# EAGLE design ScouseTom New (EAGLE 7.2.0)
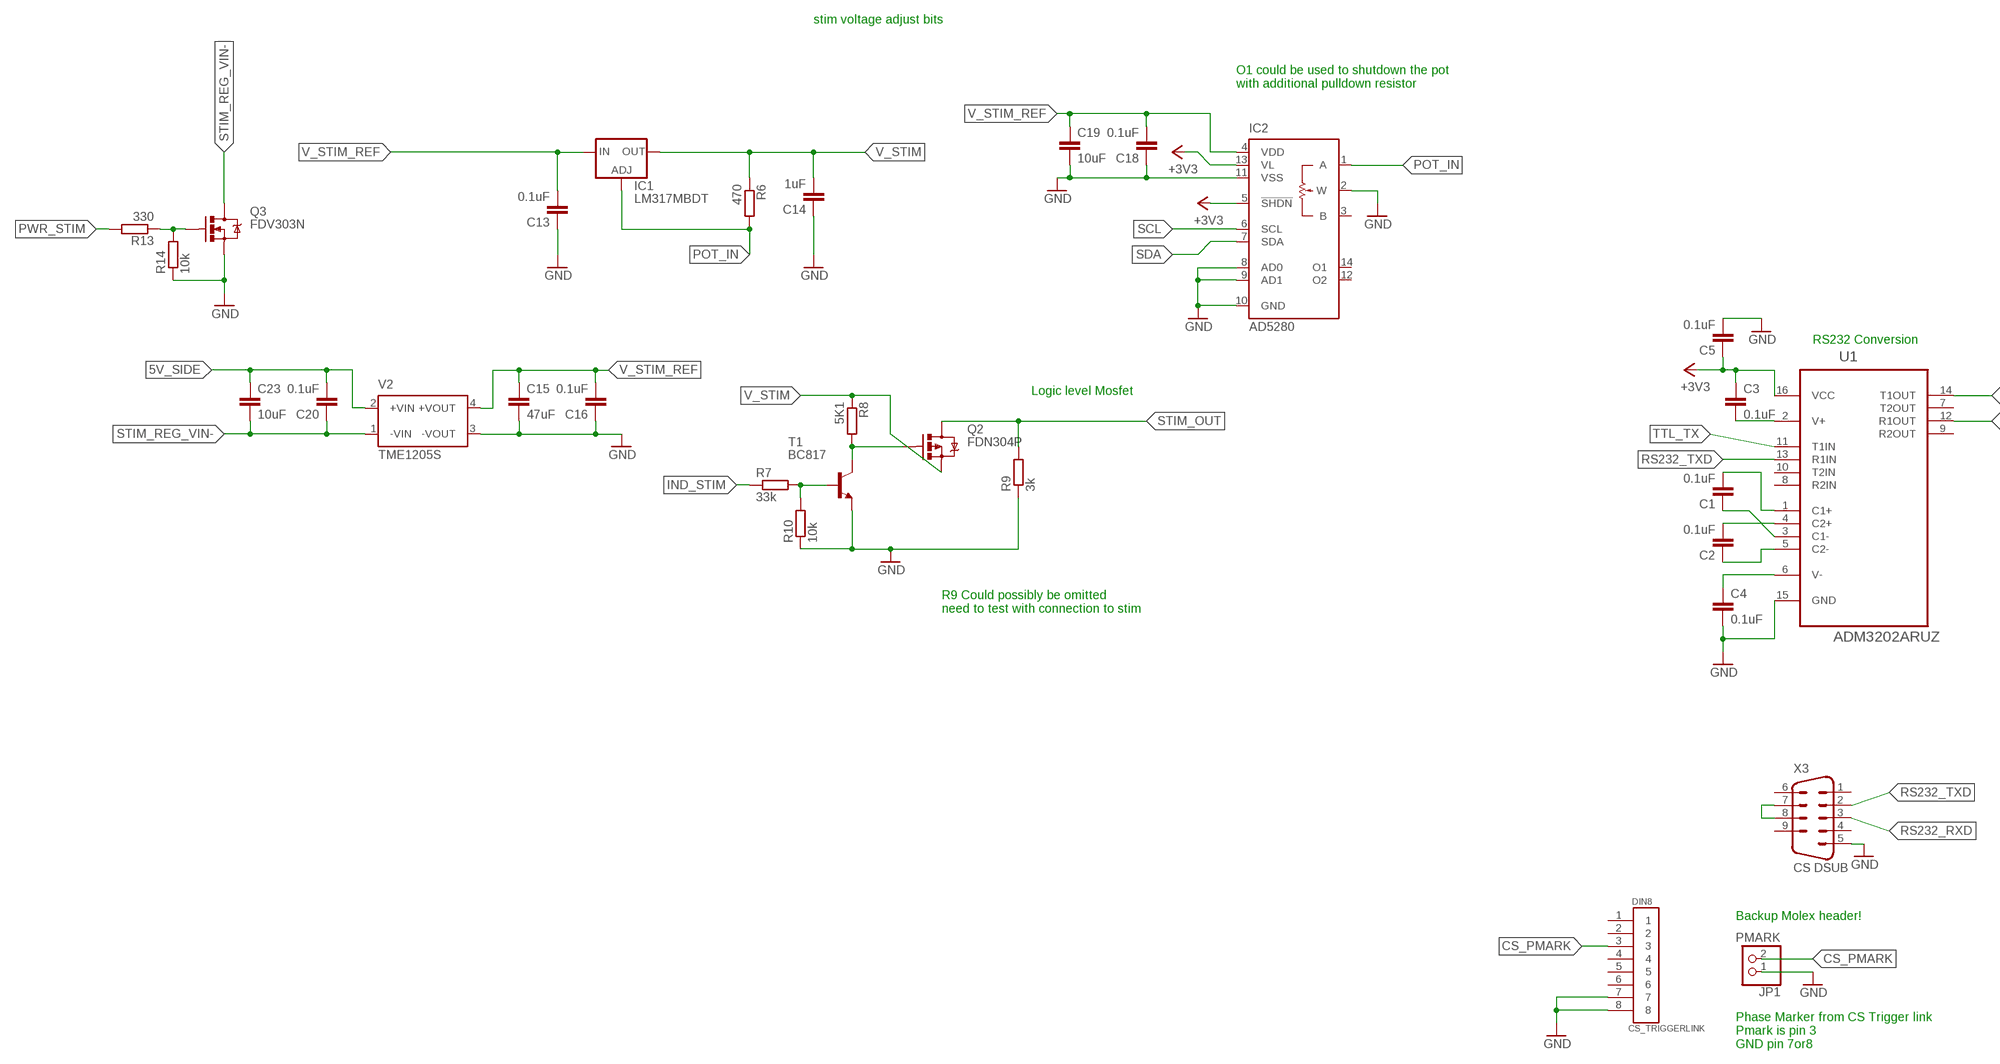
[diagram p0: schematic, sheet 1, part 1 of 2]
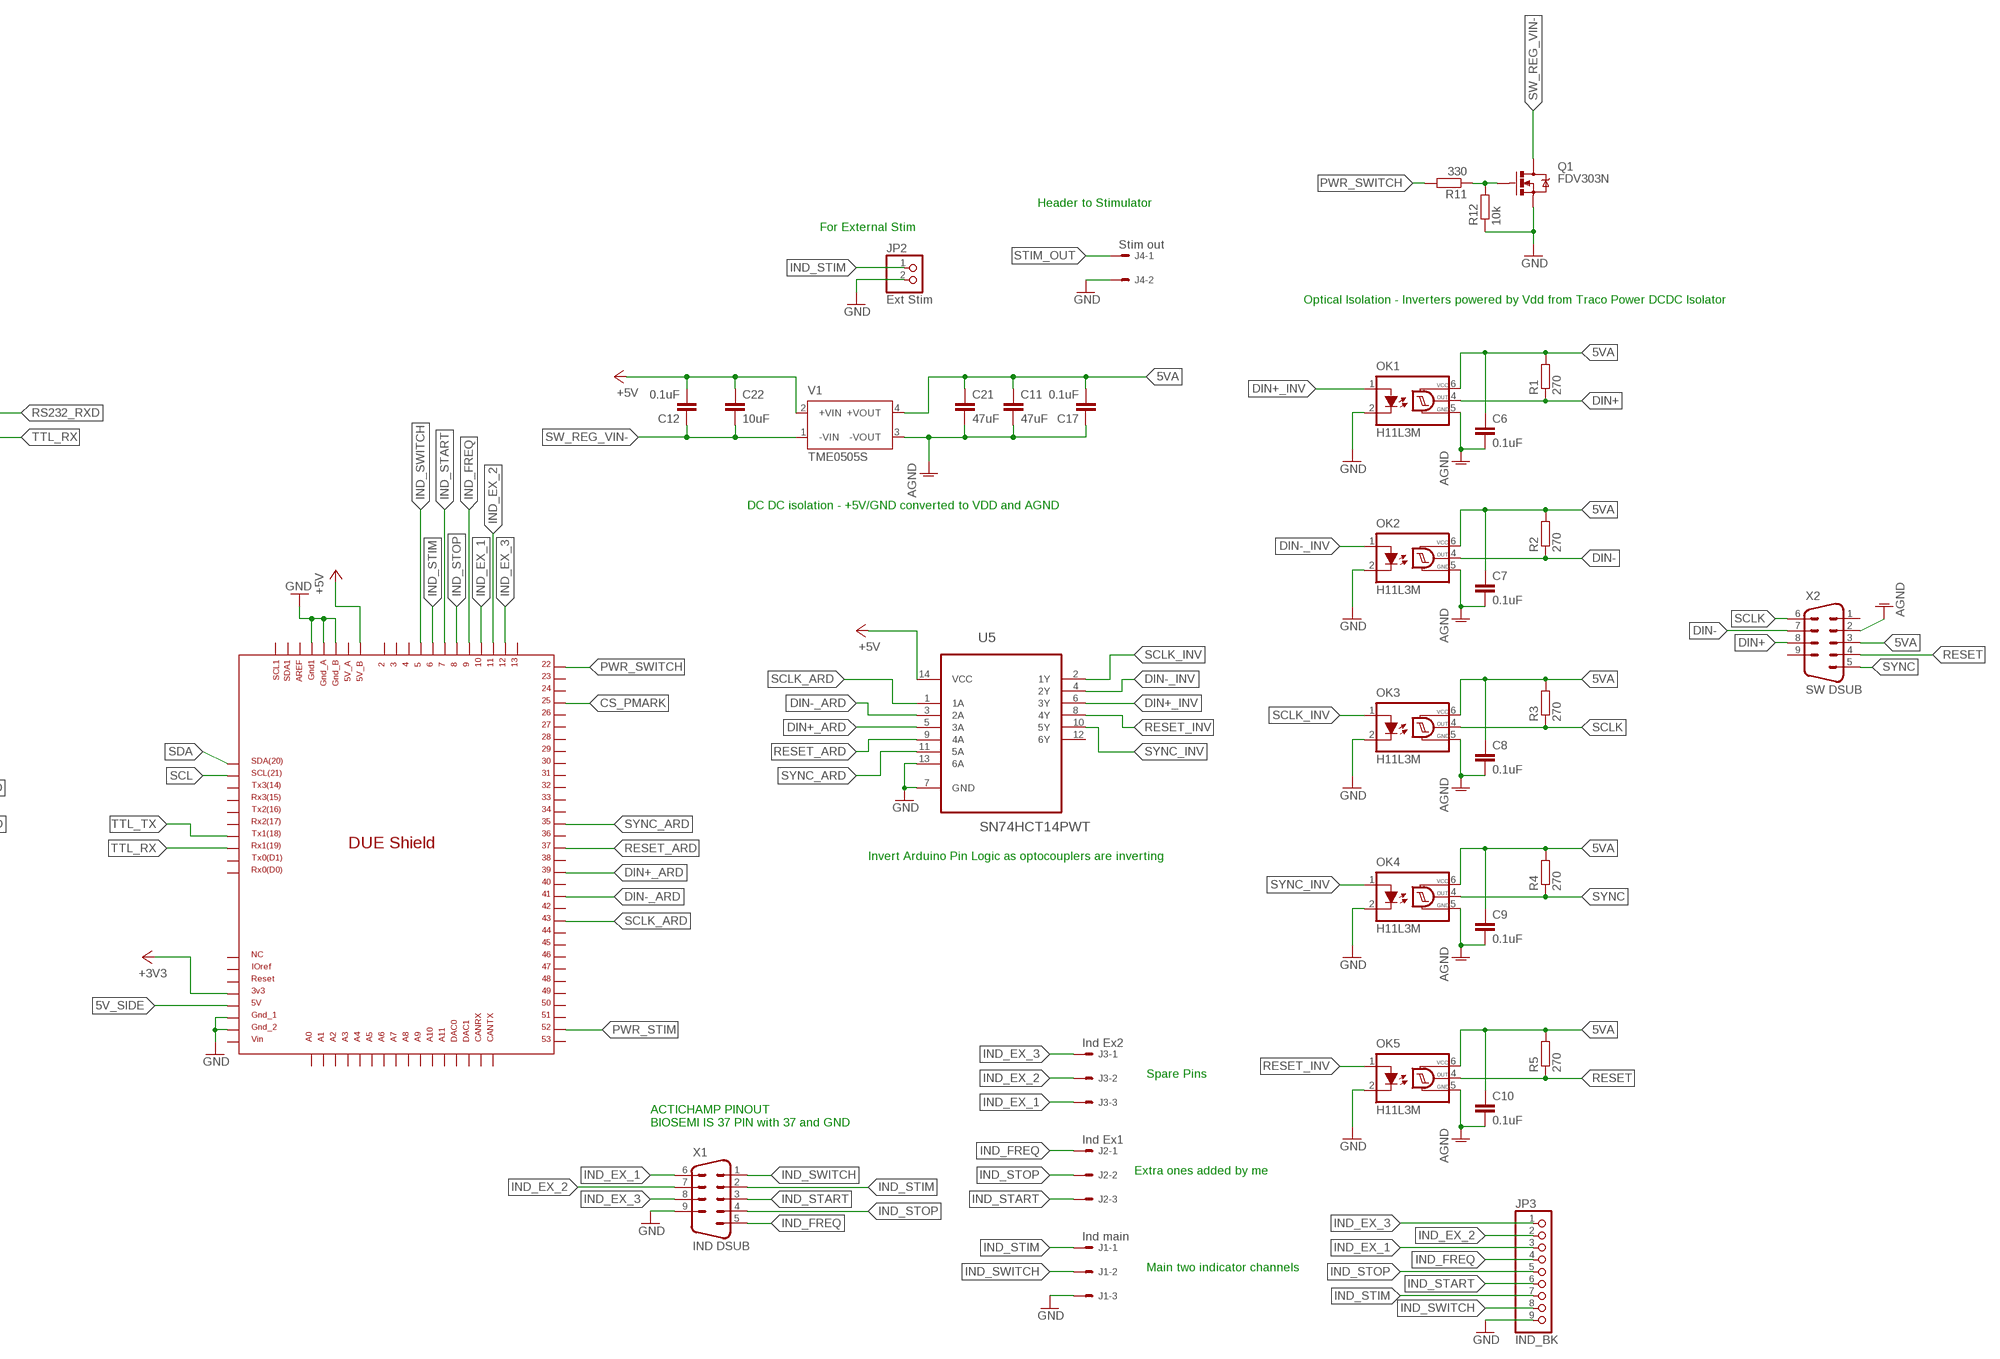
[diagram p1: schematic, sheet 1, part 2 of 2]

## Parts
C1  0.1uF  C-EUC0805  [C0805]
C2  0.1uF  C-EUC0805  [C0805]
C3  0.1uF  C-EUC0805  [C0805]
C4  0.1uF  C-EUC0805  [C0805]
C5  0.1uF  C-EUC0805  [C0805]
C6  0.1uF  C-EUC0805  [C0805]
C7  0.1uF  C-EUC0805  [C0805]
C8  0.1uF  C-EUC0805  [C0805]
C9  0.1uF  C-EUC0805  [C0805]
C10  0.1uF  C-EUC0805  [C0805]
C11  47uF  C-EUC0805  [C0805]
C12  0.1uF  C-EUC0805  [C0805]
C13  0.1uF  C-EUC0805  [C0805]
C14  1uF  C-EUC0805  [C0805]
C15  47uF  C-EUC0805  [C0805]
C16  0.1uF  C-EUC0805  [C0805]
C17  0.1uF  C-EUC0805  [C0805]
C18  0.1uF  C-EUC0805  [C0805]
C19  10uF  C-EUC0805  [C0805]
C20  0.1uF  C-EUC0805  [C0805]
C21  47uF  C-EUC0805  [C0805]
C22  10uF  C-EUC0805  [C0805]
C23  10uF  C-EUC0805  [C0805]
DIN8  CS_TRIGGERLINK  DIN8  [DIN8]
DUE  DUE(NOMID)  [DUE(NOMID)]
IC1  LM317MBDT  [DPACK]
IC2  AD5280  [TSSOP14]
J1  Ind main  22-27-2031-03  [6410-03]
J2  Ind Ex1  22-27-2031-03  [6410-03]
J3  Ind Ex2  22-27-2031-03  [6410-03]
J4  Stim out  22-27-2021-02  [6410-02]
JP1  PMARK  PINHD-1X2  [1X02]
JP2  Ext Stim  PINHD-1X2  [1X02]
JP3  IND_BK  PINHD-1X9  [1X09]
OK1  H11L3M  [DIL06]
OK2  H11L3M  [DIL06]
OK3  H11L3M  [DIL06]
OK4  H11L3M  [DIL06]
OK5  H11L3M  [DIL06]
Q1  FDV303N  MOSFET-NCHANNEL2N7002PW  [SOT323]
Q2  FDN304P  MOSFET-PCHANNEL  [SOT23-3]
Q3  FDV303N  MOSFET-NCHANNEL2N7002PW  [SOT323]
R1  270  R-EU_R0805  [R0805]
R2  270  R-EU_R0805  [R0805]
R3  270  R-EU_R0805  [R0805]
R4  270  R-EU_M0805  [M0805]
R5  270  R-EU_M0805  [M0805]
R6  470  R-EU_R0805  [R0805]
R7  33k  R-EU_R0805  [R0805]
R8  5K1  R-EU_R0805  [R0805]
R9  3k  R-EU_R0805  [R0805]
R10  10k  R-EU_R0805  [R0805]
R11  330  R-EU_R0805  [R0805]
R12  10k  R-EU_R0805  [R0805]
R13  330  R-EU_R0805  [R0805]
R14  10k  R-EU_R0805  [R0805]
T1  BC817  BC817-40SMD  [SOT23-BEC]
U1  ADM3202ARUZ  [SOP65P640X120-16N]
U5  SN74HCT14PWT  [SOP65P640X120-14N]
V1  TME0505S  [TME]
V2  TME1205S  [TME]
X1  IND DSUB  DSUB9RA  [DSUB9]
X2  SW DSUB  DSUB9RA  [DSUB9]
X3  CS DSUB  DSUB9RA  [DSUB9]

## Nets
5V_SIDE: C20.2 C23.1 DUE.5V V2.2(+VIN)
5VA: C6.1 C7.1 C8.1 C9.1 C10.1 C11.1 C17.2 C21.1 OK1.6(VCC) OK2.6(VCC) OK3.6(VCC) OK4.6(VCC) OK5.6(VCC) R1.2 R2.2 R3.2 R4.2 R5.2 V1.4(+VOUT) X2.3
+3V3: C3.1 C5.1 DUE.3V3 IC2.5(!SHDN) IC2.13(VL) U1.16(VCC)
+5V: C12.2 C22.1 DUE.5V_B U5.14(VCC) V1.2(+VIN)
AGND: C6.2 C7.2 C8.2 C9.2 C10.2 C11.2 C17.1 C21.2 OK1.5(GND) OK2.5(GND) OK3.5(GND) OK4.5(GND) OK5.5(GND) V1.3(-VOUT) X2.2
CS_PMARK: DIN8.3 DUE.25 JP1.2
DIN+: OK1.4(OUT) R1.1 X2.8
DIN+_ARD: DUE.39 U5.5(3A)
DIN+_INV: OK1.1(A) U5.6(3Y)
DIN-: OK2.4(OUT) R2.1 X2.7
DIN-_ARD: DUE.41 U5.3(2A)
DIN-_INV: OK2.1(A) U5.4(2Y)
GND: C4.2 C5.2 C13.1 C14.1 C15.2 C16.1 C18.1 C19.2 DIN8.7 DIN8.8 DUE.GND1 DUE.GND_1 DUE.GND_2 DUE.GND_A DUE.GND_B IC2.2(W) IC2.8(AD0) IC2.9(AD1) IC2.10(GND) IC2.11(VSS) J1.3 J4.2 JP1.1 JP2.2 JP3.9 OK1.2(C) OK2.2(C) OK3.2(C) OK4.2(C) OK5.2(C) Q1.2(S) Q3.2(S) R9.1 R10.1 R12.1 R14.1 T1.E U1.15(GND) U5.7(GND) U5.13(6A) V2.3(-VOUT) X1.9 X3.5
IND_EX_1: DUE.10 J3.3 JP3.3 X1.6
IND_EX_2: DUE.11 J3.2 JP3.2 X1.7
IND_EX_3: DUE.12 J3.1 JP3.1 X1.8
IND_FREQ: DUE.9 J2.1 JP3.4 X1.5
IND_START: DUE.7 J2.3 JP3.6 X1.3
IND_STIM: DUE.6 J1.1 JP2.1 JP3.7 R7.1 X1.2
IND_STOP: DUE.8 J2.2 JP3.5 X1.4
IND_SWITCH: DUE.5 J1.2 JP3.8 X1.1
N$1: R7.2 R10.2 T1.B
N$2: Q1.1(G) R11.1 R12.2
N$3: Q2.1(G) R8.2 T1.C
N$4: X3.7 X3.8
N$5: Q3.1(G) R13.1 R14.2
N$22: C1.2 U1.1(C1+)
N$23: C1.1 U1.3(C1-)
N$24: C2.2 U1.4(C2+)
N$25: C2.1 U1.5(C2-)
N$26: C3.2 U1.2(V+)
N$27: C4.1 U1.6(V-)
POT_IN: IC1.1(ADJ) IC2.1(A) R6.2
PWR_STIM: DUE.52 R13.2
PWR_SWITCH: DUE.22 R11.2
RESET: OK5.4(OUT) R5.1 X2.4
RESET_ARD: DUE.37 U5.9(4A)
RESET_INV: OK5.1(A) U5.8(4Y)
RS232_RXD: U1.14(T1OUT) X3.3
RS232_TXD: U1.13(R1IN) X3.2
SCL: DUE.SCL IC2.6(SCL)
SCLK: OK3.4(OUT) R3.1 X2.6
SCLK_ARD: DUE.43 U5.1(1A)
SCLK_INV: OK3.1(A) U5.2(1Y)
SDA: DUE.SDA IC2.7(SDA)
STIM_OUT: J4.1 Q2.3(D) R9.2
STIM_REG_VIN-: C20.1 C23.2 Q3.3(D) V2.1(-VIN)
SW_REG_VIN-: C12.1 C22.2 Q1.3(D) V1.1(-VIN)
SYNC: OK4.4(OUT) R4.1 X2.5
SYNC_ARD: DUE.35 U5.11(5A)
SYNC_INV: OK4.1(A) U5.10(5Y)
TTL_RX: DUE.RX1 U1.12(R1OUT)
TTL_TX: DUE.TX1 U1.11(T1IN)
V_STIM: C14.2 IC1.4(OUT) Q2.2(S) R6.1 R8.1
V_STIM_REF: C13.2 C15.1 C16.2 C18.2 C19.1 IC1.3(IN) IC2.4(VDD) V2.4(+VOUT)
Unconnected: DIN8.1 DIN8.2 DIN8.4 DIN8.5 DIN8.6 DUE.2 DUE.3 DUE.4 DUE.5V_A DUE.13 DUE.23 DUE.24 DUE.26 DUE.27 DUE.28 DUE.29 DUE.30 DUE.31 DUE.32 DUE.33 DUE.34 DUE.36 DUE.38 DUE.40 DUE.42 DUE.44 DUE.45 DUE.46 DUE.47 DUE.48 DUE.49 DUE.50 DUE.51 DUE.53 DUE.A0 DUE.A1 DUE.A2 DUE.A3 DUE.A4 DUE.A5 DUE.A6 DUE.A7 DUE.A8 DUE.A9 DUE.A10 DUE.A11 DUE.AREF DUE.CANRX DUE.CANTX DUE.DAC0 DUE.DAC1 DUE.IOREF DUE.NC DUE.RESET DUE.RX0 DUE.RX2 DUE.RX3 DUE.SCL1 DUE.SDA1 DUE.TX0 DUE.TX2 DUE.TX3 DUE.VIN IC2.3(B) IC2.12(O2) IC2.14(O1) U1.7(T2OUT) U1.8(R2IN) U1.9(R2OUT) U1.10(T2IN) U5.12(6Y) X2.1 X2.9 X3.1 X3.4 X3.6 X3.9

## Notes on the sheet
- stim voltage adjust bits
- O1 could be used to shutdown the pot
  with additional pulldown resistor
- Header to Stimulator
- For External Stim
- Optical Isolation - Inverters powered by Vdd from Traco Power DCDC Isolator
- RS232 Conversion
- Logic level Mosfet
- DC DC isolation - +5V/GND converted to VDD and AGND
- R9 Could possibly be omitted
  need to test with connection to stim
- Invert Arduino Pin Logic as optocouplers are inverting
- Backup Molex header!
- Phase Marker from CS Trigger link
  Pmark is pin 3
  GND pin 7or8
- Spare Pins
- ACTICHAMP PINOUT
  BIOSEMI IS 37 PIN with 37 and GND
- Extra ones added by me
- Main two indicator channels

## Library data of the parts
C1-C23 = resistor:C-EU: CAPACITOR, European symbol
DIN8 = mini din 8 james:DIN8
DUE = DUElib130425_JAMES:DUE(NOMID)
IC1 = v-reg:LM317?*: 500 mA Adjustable Output Positive Voltage Regulator Source: http://www.onsemi.co.jp .. LM317M-D.PDF
IC2 = analog-devices:AD5280: Single +15 V/±5 V, 256-Position, I2C-Compatible Digital Potentiometer Source: http://www.analog.com/static/imported-files/data_sheets/AD5280_5282.pdf; MF: ALTERA CORPORATION; MPN: AD5280BRUZ20; OC_FARNELL: 1464325; OC_NEWARK: 59K3840
J1-J3 = con-molex:22-?-03: CONNECTOR wire to board 2.54 mm (.1 inch) pitch header; OC_FARNELL: unknown; OC_NEWARK: unknown
J4 = con-molex:22-?-02: CONNECTOR; OC_FARNELL: unknown; OC_NEWARK: unknown
JP1 JP2 = pinhead:PINHD-1X2: PIN HEADER
JP3 = pinhead:PINHD-1X9: PIN HEADER
OK1-OK5 = optocoupler:H11L*M: 6-Pin DIP Optocoupler Source: http://www.fairchildsemi.com/ds/H1/H11L2-M.pdf; MF: FAIRCHILD SEMICONDUCTOR; MPN: H11L3-M; OC_FARNELL: 1021233; OC_NEWARK: 72K8646
Q1 Q3 = SparkFun-DiscreteSemi:MOSFET-NCHANNEL: Common NMOSFET Parts MFG P/NStore IDProd ID FDD8780TRANS-09984 SI7820DNTRANS-11055 FDS6630AIC-08089 2N7002PWTRANS-11151 FQP30N06L COM-10213TRANS-10060 BSS123LT1GTRANS-08345 BSS138TRANS-00830 BS170 2N7000; PROD_ID: TRANS-11151
Q2 = SparkFun-DiscreteSemi:MOSFET-PCHANNEL: Generic PMOSFET IRLML2244 - TRANS-11153 (SOT-23 -20V -4.3A) (1.Gate 2.Source 3.Drain) FQP27P06 - COM-10349 (TO-220 -60V -27A) (1.Gate 2.Source 3.Drain); PROD_ID: TRANS-08285
R1-R14 = resistor:R-EU_: RESISTOR, European symbol
T1 = transistor-npn:BC817*: NPN Transistor
U1 = Analog Devices_By_element14_Batch_1:ADM3202ARUZ: Low Power, 3.3 V, RS-232 Line Drivers/Receivers; MPN: ADM3202ARUZ; OC_FARNELL: 9425586; OC_NEWARK: 59K2064; PACKAGE: TSSOP-16; SUPPLIER: Analog Devices
U5 = untitled:SN74HCT14PWT: QUADRUPLE FET BUS SWITCH 2.5-V/3.3-V LOW-VOLTAGE BUS SWITCH WITH 5-V-TOLERANT LEVEL SHIFTER; MPN: SN74HCT14PWT; OC_FARNELL: 1236233; OC_NEWARK: 13M5201; PACKAGE: TSSOP-14; SUPPLIER: Texas Instruments
V1 = traco-electronic:TME?*: DC/DC Converter TME Series 1 Watt Source: www.tracopower.com .. tme.pdf; MPN: TME 0505S; OC_FARNELL: 1007538; OC_NEWARK: 51R5321
V2 = traco-electronic:TME?*: DC/DC Converter TME Series 1 Watt Source: www.tracopower.com .. tme.pdf; MPN: TME 1205S; OC_FARNELL: 1007542; OC_NEWARK: 51R5325
X1-X3 = DSUBJAMES:DSUB9RA

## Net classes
1 power: width 0.61 mm, drill 0.61 mm, clearance 0.254 mm
2 gnd: width 0.305 mm, drill 0.559 mm, clearance 0.254 mm
3 usbvcc: width 0.508 mm, drill 0.61 mm, clearance 0.254 mm
4 aref: width 0.406 mm, drill 0.61 mm, clearance 0.254 mm

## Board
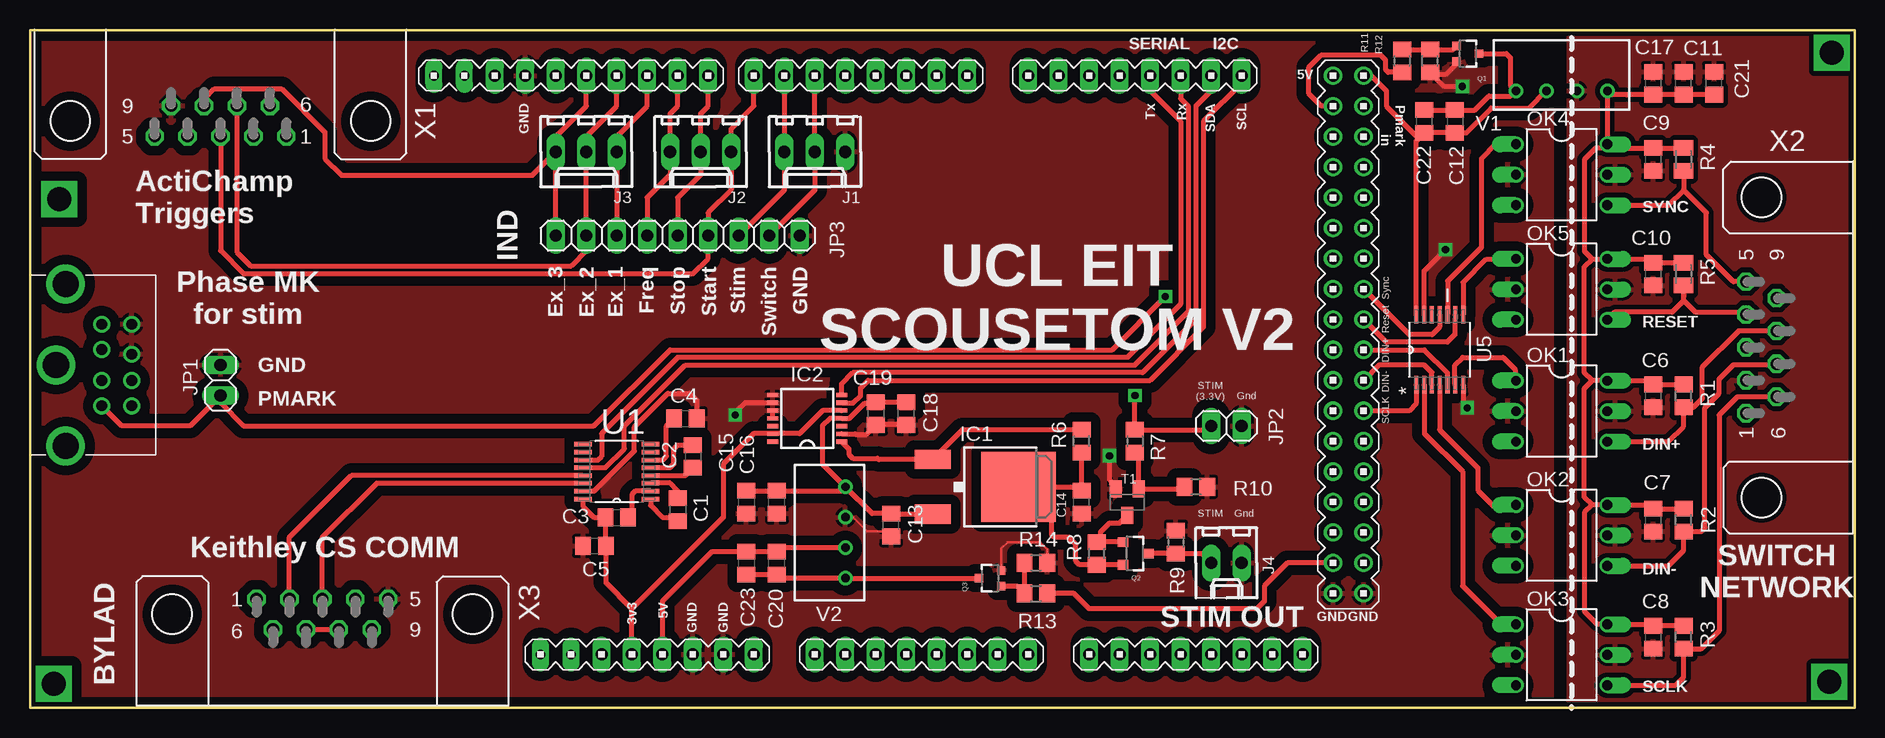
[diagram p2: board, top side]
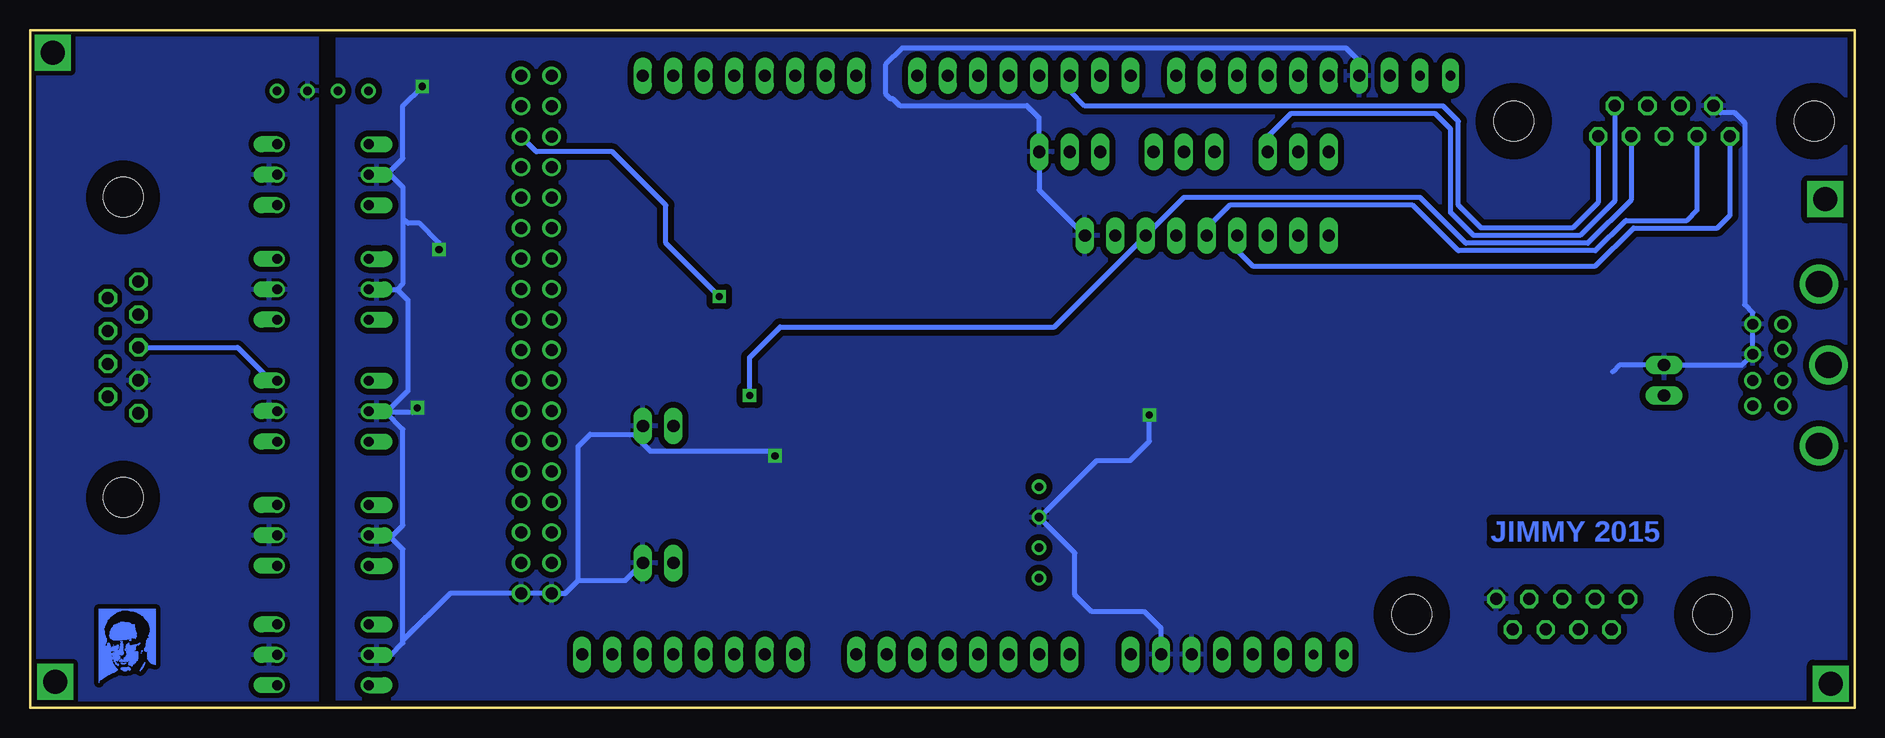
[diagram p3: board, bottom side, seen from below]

Size 152.05 x 56.52 mm. Coordinates in mm from the lower left corner, seen from the top.
Outline: 152.05,56.52 0,56.52 0,0 152.05,0 152.05,56.52
Copper layers (1*16): Top 0.035mm / dielectric 1.5mm / Bottom 0.035mm
Design rules "pcbtrain": minimum track width 0.2mm, minimum drill 0.4mm, track to track 0.2mm, track to pad 0.2mm, pad to pad 0.2mm, via to via 0.2mm, smd to smd 0mil, copper to edge 10mil, drill to drill 0.2mm, minimum pad ring 10mil, minimum via ring 10mil, stop-mask expansion 0.125mm, vias tented up to drill 0mil, thermal gap 10mil

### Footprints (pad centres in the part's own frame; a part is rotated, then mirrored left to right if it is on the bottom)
C0805 = smd 1.3 x 1.5: 1 -0.95,0; 2 0.95,0
DIN8 = drill 0.9: 1 -1.3,-3.8; 2 1.3,-3.8; 3 -3.4,-3.8; 4 -1.3,-6.3; 5 3.4,-3.8; 6 -3.4,-6.3; 7 0.9,-6.3; 8 3.4,-6.3 | drill 2.2: P$1 0,0; P$2 -6.75,-0.8; P$3 6.75,-0.8
DUE(NOMID) = drill 1 long: 2 -5.08,25.4; 3 -7.62,25.4; 3V3 -27.94,-22.86; 4 -10.16,25.4; 5 -12.7,25.4; 5V -25.4,-22.86; 6 -15.24,25.4; 7 -17.78,25.4; 8 -21.59,25.4; 9 -24.13,25.4; 10 -26.67,25.4; 11 -29.21,25.4; 12 -31.75,25.4; 13 -34.29,25.4; A0 -12.7,-22.86; A1 -10.16,-22.86; A2 -7.62,-22.86; A3 -5.08,-22.86; A4 -2.54,-22.86; A5 0,-22.86; A6 2.54,-22.86; A7 5.08,-22.86; A8 10.16,-22.86; A9 12.7,-22.86; A10 15.24,-22.86; A11 17.78,-22.86; AREF -39.37,25.4; CANRX 25.4,-22.86; CANTX 27.94,-22.86; DAC0 20.32,-22.86; DAC1 22.86,-22.86; GND1 -36.83,25.4; GND_1 -22.86,-22.86; GND_2 -20.32,-22.86; RESET -30.48,-22.86; RX0 0,25.4; RX1 17.78,25.4; RX2 12.7,25.4; RX3 7.62,25.4; SCL 22.86,25.4; SDA 20.32,25.4; TX0 -2.54,25.4; TX1 15.24,25.4; TX2 10.16,25.4; TX3 5.08,25.4; VIN -17.78,-22.86 | drill 1: 5V_A 30.48,25.4; 5V_B 33.02,25.4; 22 30.48,22.86; 23 33.02,22.86; 24 30.48,20.32; 25 33.02,20.32; 26 30.48,17.78; 27 33.02,17.78; 28 30.48,15.24; 29 33.02,15.24; 30 30.48,12.7; 31 33.02,12.7; 32 30.48,10.16; 33 33.02,10.16; 34 30.48,7.62; 35 33.02,7.62; 36 30.48,5.08; 37 33.02,5.08; 38 30.48,2.54; 39 33.02,2.54; 40 30.48,0; 41 33.02,0; 42 30.48,-2.54; 43 33.02,-2.54; 44 30.48,-5.08; 45 33.02,-5.08; 46 30.48,-7.62; 47 33.02,-7.62; 48 30.48,-10.16; 49 33.02,-10.16; 50 30.48,-12.7; 51 33.02,-12.7; 52 30.48,-15.24; 53 33.02,-15.24; GND_A 30.48,-17.78; GND_B 33.02,-17.78 | drill 0.8 pad 1.422 long: IOREF -33.02,-22.86; NC -35.56,-22.86; SCL1 -44.45,25.4; SDA1 -41.91,25.4
DPACK = smd 1.6 x 3: 1 -2.28,-4.8; 3 2.28,-4.8 | smd 5.8 x 6.2: 4 0,2.38
TSSOP14 = smd 0.9 x 0.35: 1 -2.875,1.95; 2 -2.875,1.3; 3 -2.875,0.65; 4 -2.875,0; 5 -2.875,-0.65; 6 -2.875,-1.3; 7 -2.875,-1.95; 8 2.875,-1.95; 9 2.875,-1.3; 10 2.875,-0.65; 11 2.875,0; 12 2.875,0.65; 13 2.875,1.3; 14 2.875,1.95
6410-03 = drill 1.016 long: 1 2.54,0; 2 0,0; 3 -2.54,0
6410-02 = drill 1.016 long: 1 1.27,0; 2 -1.27,0
1X02 = drill 1.016 long: 1 -1.27,0; 2 1.27,0
1X09 = drill 1.016 long: 1 -10.16,0; 2 -7.62,0; 3 -5.08,0; 4 -2.54,0; 5 0,0; 6 2.54,0; 7 5.08,0; 8 7.62,0; 9 10.16,0
DIL06 = drill 0.813 offset: 1 -2.54,-3.81; 2 0,-3.81; 3 2.54,-3.81; 4 2.54,3.81; 5 0,3.81; 6 -2.54,3.81
SOT323 = smd 0.7 x 0.7: 1 -0.65,-0.925; 2 0.65,-0.925; 3 0,0.925
SOT23-3 = smd 0.8 x 0.9: 1 -0.95,-1; 2 0.95,-1; 3 0,1.1
R0805 = smd 1.3 x 1.5: 1 -0.95,0; 2 0.95,0
M0805 = smd 1.3 x 1.6: 1 -0.95,0; 2 0.95,0
SOT23-BEC = smd 1 x 1.4: B -0.95,-1.1; C 0,1.1; E 0.95,-1.1
SOP65P640X120-16N = smd 1.473 x 0.356: 1 -2.819,2.286; 2 -2.819,1.626; 3 -2.819,0.965; 4 -2.819,0.33; 5 -2.819,-0.33; 6 -2.819,-0.965; 7 -2.819,-1.626; 8 -2.819,-2.286; 9 2.819,-2.286; 10 2.819,-1.626; 11 2.819,-0.965; 12 2.819,-0.33; 13 2.819,0.33; 14 2.819,0.965; 15 2.819,1.626; 16 2.819,2.286
SOP65P640X120-14N = smd 1.473 x 0.356: 1 -2.921,1.956; 2 -2.921,1.295; 3 -2.921,0.66; 4 -2.921,0; 5 -2.921,-0.66; 6 -2.921,-1.295; 7 -2.921,-1.956; 8 2.921,-1.956; 9 2.921,-1.295; 10 2.921,-0.66; 11 2.921,0; 12 2.921,0.66; 13 2.921,1.295; 14 2.921,1.956
TME = drill 0.7 pad 1.1: 1 -3.81,0; 2 -1.27,0; 3 1.27,0; 4 3.81,0
DSUB9 = drill 1.016 octagon: 1 -5.486,0; 2 -2.743,0; 3 0,0; 4 2.743,0; 5 5.486,0; 6 -4.115,-2.54; 7 -1.372,-2.54; 8 1.372,-2.54; 9 4.115,-2.54 | hole 3.302: 12.522,-1.27; -12.522,-1.27

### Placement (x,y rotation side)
C1  53.98,16.51 270 top
C2  55.25,20.95 270 top
C3  48.89,15.88 0 top
C4  54.61,24.13 0 top
C5  47.03,13.47 180 top
C6  135.25,26 270 top
C7  135.25,15.64 270 top
C8  135.25,5.88 270 top
C9  135.25,45.72 270 top
C10  135.25,36.16 270 top
C11  137.8,52.07 90 top
C12  118.75,48.89 270 top
C13  71.75,15.24 90 top
C14  87.63,17.15 90 top
C15  59.69,17.15 270 top
C16  62.23,17.15 90 top
C17  135.25,52.07 270 top
C18  73.03,24.53 90 top
C19  70.48,24.53 270 top
C20  62.23,12.06 90 top
C21  140.33,52.07 90 top
C22  116.2,48.89 90 top
C23  59.69,12.06 270 top
DIN8  2.18,28.57 90 top
DUE  78.11,27.3 0 top
IC1  80.01,18.41 270 top
IC2  64.77,24.13 180 top
J1  65.41,46.35 180 top
J2  55.88,46.35 180 top
J3  46.36,46.35 180 top
J4  99.7,12.06 180 top
JP1  15.88,27.3 270 top
JP2  99.7,23.49 0 top
JP3  53.98,39.37 0 top
OK1  127.64,24.73 270 top
OK2  127.64,14.37 270 top
OK3  127.64,4.41 270 top
OK4  127.64,44.45 270 top
OK5  127.64,34.89 270 top
Q1  119.81,54.54 270 top
Q2  92.08,12.87 270 top
Q3  80.01,10.79 90 top
R1  137.8,26 90 top
R2  137.8,15.64 90 top
R3  137.8,5.88 90 top
R4  137.8,45.72 90 top
R5  137.8,36.16 90 top
R6  87.63,22.23 90 top
R7  92.08,22.23 270 top
R8  88.9,12.87 90 top
R9  95.48,13.81 270 top
R10  97.16,18.41 180 top
R11  114.33,53.94 270 top
R12  116.67,53.94 90 top
R13  83.82,9.53 0 top
R14  83.82,12.06 180 top
T1  91.44,17.15 180 top
U1  48.89,19.69 180 top
U5  117.47,29.84 90 top
V1  127.64,51.43 0 top
V2  67.94,14.6 90 top
X1  15.88,47.65 180 top
X2  143.01,30.05 90 top
X3  24.37,9.06 0 top

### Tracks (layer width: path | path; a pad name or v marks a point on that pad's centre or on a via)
5V_SIDE
  Top 0.406: DUE.5V 52.7,8.89 56.83,13.01 C23.1 C20.2 62.55,13.33 V2.2
5VA
  Top 0.406: C21.1 C11.1 C17.2 133.03,51.12 131.76,51.12 V1.4 OK4.6 131.76,46.67 | 131.76,46.67 C9.1 R4.2 | R5.2 C10.1 134.94,37.43 OK5.6 130.18,37.43 | 131.76,46.67 130.49,46.67 129.54,45.72 129.54,38.06 130.18,37.43 | 130.18,27.27 OK1.6 134.94,27.27 C6.1 R1.2 | 130.18,27.27 129.54,27.91 129.54,36.8 130.18,37.43 | 130.18,16.91 129.54,17.55 129.54,26.63 130.18,27.27 | 130.18,16.91 OK2.6 134.94,16.91 C7.1 R2.2 | 130.18,16.91 129.54,16.27 129.54,8.03 130.56,7.01 131.39,7.01 OK3.6 135.13,6.95 C8.1 R3.2
  Bottom 0.406: X2.3 134.74,30.05 131.97,27.27 OK1.6
+3V3
  Top 0.406: IC2.5 66.06,24.78 64.13,22.86 61.92,22.86 | 61.92,22.86 IC2.13 | U1.16 46.08,16.79 46.99,15.88 C3.1 47.95,13.51 C5.1 47.98,10.44 50.16,8.26 | 61.92,22.86 60.33,22.86 57.79,20.32 57.79,15.88 50.16,8.26 | DUE.3V3 50.16,8.26
+5V
  Top 0.406: U5.14 115.52,47.26 115.73,47.47 | 115.73,47.47 C22.1 C12.2 119.7,47.95 121.77,50 124.94,50 V1.2 | DUE.5V_B 111.76,52.7 113.03,51.43 113.03,50.16 115.73,47.47
AGND
  pour Top (isolate 0.406): 128.27,56.52 152.05,56.52 152.05,0 128.27,0
  pour Bottom (isolate 0.4): 128.17,56.41 151.97,56.41 151.97,0.01 128.17,0.01
CS_PMARK  (via drill 0.6)
  Top 0.406: v94.61,34.29 90.17,29.84 53.34,29.84 46.99,23.49 17.78,23.49 15.88,25.4 JP1.2 13.34,23.49 7.66,23.49 DIN8.3
  Bottom 0.406: v94.61,34.29 99.06,38.73 99.06,41.91 103.5,46.35 109.86,46.35 DUE.25
DIN+
  Top 0.406: OK1.4 136.53,22.19 137.8,23.46 R1.1 138.61,25.05 139.37,25.8 139.37,28.41 142.38,31.42 X2.8
DIN+_ARD
  Top 0.406: DUE.39 116.2,29.84 118.11,27.94 118.11,26.95 U5.5
DIN+_INV
  Top 0.406: U5.6 118.75,26.95 118.75,28.57 119.38,29.21 122.76,29.21 123.77,28.2 123.77,27.33 OK1.1
DIN-
  Top 0.406: OK2.4 136.53,11.83 137.8,13.1 R2.1 139.25,14.69 139.56,15.01 139.56,25 140.76,26.2 140.76,27.41 141.97,28.6 145.49,28.6 X2.7
DIN-_ARD
  Top 0.406: U5.3 116.81,27.96 116.2,28.57 112.39,28.57 DUE.41
DIN-_INV
  Top 0.406: U5.4 117.47,23.18 120.65,20 120.65,18.12 121.97,16.8 123.72,16.8 OK2.1
GND  (via drill 0.6)
  Top 0.2: V2.3 68.59,15.88 69.77,14.71 71.34,14.71 C13.1 | Q3.2 80.94,13.28 81.47,13.81 84.16,13.81 84.77,13.21 R14.1
  Top 0.406: IC2.2 68.74,22.83 68.77,22.8 69.71,22.8 C19.2 70.51,23.6 72.97,23.6 72.99,23.58 C18.1 | U5.13 116.18,36.42 v117.97,38.2 | v119.36,51.8 117.86,51.8 R12.1 116.86,52.8 117.97,52.8 118.89,53.73 Q1.2 | v58.77,24.41 58.77,24.6 59.59,25.43 IC2.9 | T1.E 90.17,18.57 90.17,18.8 89.97,19.01 v89.97,21.01 | U1.15 47.02,18.06 50.37,21.41 50.37,23.41 53.16,26.2 54.97,26.2 55.56,25.6 C4.2 | U5.7 119.43,25.34 v119.77,25 | IC2.11 IC2.10
  Bottom 0.406: OK3.2 121.96,4.41 120.97,5.4 120.97,5.6 | 120.97,5.6 120.97,13.21 122.13,14.37 OK2.2 121.8,14.37 120.97,15.21 120.97,23.2 122.36,24.6 | 122.36,24.6 123.7,24.6 OK1.2 | OK5.2 121.45,34.89 | 121.45,34.89 120.56,34 120.56,26.41 122.36,24.6 | OK4.2 122.01,44.45 | 122.01,44.45 120.97,43.41 120.97,40.8 | 120.97,40.8 120.97,35.38 121.45,34.89 | 106.36,10.6 107.45,9.53 DUE.GND_A DUE.GND_B 117.05,9.53 120.97,5.6 | 106.36,10.6 106.36,21.8 105.36,22.8 101.66,22.8 | 101.66,22.8 JP2.2 | 106.36,10.6 102.42,10.6 J4.2 | 20.16,28 19.59,28.57 JP1.1 9.38,28.57 DIN8.7 DIN8.8 8.48,32.91 9.17,33.6 9.17,48.8 9.96,49.6 11.18,49.6 X1.9 | DUE.GND1 41.28,53.91 42.37,55 79.37,55 80.77,53.61 80.77,51.2 80.37,50.8 80.16,50.8 79.56,50.2 68.97,50.2 67.97,49.2 67.97,46.38 J1.3 67.94,43.18 JP3.9 | DUE.GND_2 57.79,6.63 59.16,8.01 63.56,8.01 64.97,9.4 64.97,12.9 V2.3 67.9,15.88 63.16,20.6 60.37,20.6 58.77,22.2 v58.77,24.41 | v117.97,38.2 117.97,38.8 119.56,40.41 120.56,40.41 120.97,40.8 | 122.01,44.45 122.01,44.76 120.97,45.8 120.97,50.2 v119.36,51.8 | 101.66,22.8 101.66,22.7 100.36,21.41 90.36,21.41 v89.97,21.01 | v119.77,25 120.17,24.6 122.36,24.6
  pour Top (isolate 0.813): -0.04,56.41 126.77,56.41 126.77,0.01 0.07,0.51
  pour Bottom (isolate 0.5): 0.16,56.41 0.02,0.53 126.36,0.21 126.36,56.41
IND_EX_1
  Top 0.406: DUE.10 51.44,50.16 48.89,47.62 J3.3 JP3.3
  Bottom 0.406: X1.6 19.99,42.24 22.86,39.37 31.75,39.37 33.66,41.27 33.66,48.26 34.92,49.53 46.99,49.53 48.89,47.62 J3.3
IND_EX_2
  Top 0.406: DUE.11 48.89,50.16 46.36,47.62 J3.2 JP3.2 46.36,38.1 45.09,36.83 18.41,36.83 17.25,38 X1.7
IND_EX_3
  Top 0.406: J3.1 43.81,47.62 46.36,50.16 DUE.12 | JP3.1 J3.1 | J3.1 41.87,44.41 25.96,44.41 24.57,45.8 24.57,48 20.96,51.6 15.37,51.6 14.5,50.74 X1.8
IND_FREQ
  Top 0.406: JP3.4 51.44,42.55 53.34,44.45 J2.1 53.34,49.53 53.98,50.16 DUE.9
  Bottom 0.406: JP3.4 51.44,38.1 50.16,36.83 21.59,36.83 18.41,40 11.43,40 10.39,41.05 X1.5
IND_START
  Top 0.406: DUE.7 60.33,50.16 58.42,48.26 J2.3 58.42,43.18 56.52,41.27 JP3.6 56.52,37.46 55.25,36.2 17.78,36.2 15.88,38.1 X1.3
IND_STIM  (via drill 0.6)
  Top 0.406: DUE.6 J1.1 62.87,43.18 JP3.7 | JP2.1 98.11,23.17 R7.1 v92.08,26.03
  Bottom 0.406: X1.2 18.62,42.34 22.23,38.73 32.38,38.73 36.2,42.55 55.88,42.55 JP3.7 66.67,31.75 89.53,31.75 92.08,29.21 v92.08,26.03
IND_STOP
  Top 0.406: DUE.8 56.52,50.16 55.88,49.53 J2.2 55.88,44.45 53.98,42.55 JP3.5
  Bottom 0.406: JP3.5 53.98,40 52.07,41.91 36.83,41.91 33.02,38.1 21.59,38.1 19.05,40.64 13.97,40.64 13.13,41.48 X1.4
IND_SWITCH
  Top 0.406: JP3.8 65.41,43.18 J1.2 DUE.5
  Bottom 0.406: X1.1 21.36,42.14 23.5,40 31.12,40 33.02,41.91 33.02,48.89 34.29,50.16 64.13,50.16 65.41,51.43 DUE.5
N$1
  Top 0.406: R10.2 95.56,18.24 T1.B 92.39,20.96 R7.2
N$2
  Top 0.406: R11.1 R12.2 118.59,54.89 Q1.1
N$3
  Top 0.406: Q2.1 R8.2 88.9,14.13 89.22,14.13 89.22,14.66 89.97,15.4 90.8,15.4 T1.C 91.44,15.56
N$4
  Top 0.406: X3.7 X3.8
N$5
  Top 0.406: Q3.1 82.25,10.15 R13.1 R14.2
N$6  (via drill 2)
  other vias: 149.94,2.16
N$7  (via drill 2)
  other vias: 150.17,54.61
N$8  (via drill 2)
  other vias: 2.42,42.41
N$9  (via drill 2)
  other vias: 1.96,2.01
N$22
  Top 0.406: U1.1 51.71,16.87 52.7,15.88 53.66,15.88 C1.2
N$23
  Top 0.406: C1.1 53.98,18.1 53.34,18.73 51.73,18.73 U1.3
N$24
  Top 0.406: U1.4 54.59,19.35 C2.2
N$25
  Top 0.406: U1.5 53.35,20.02 53.66,20.32 53.66,21.59 53.98,21.91 C2.1
N$26
  Top 0.406: U1.2 50.44,18.06 50.16,17.78 50.16,16.2 C3.2
N$27
  Top 0.406: U1.6 52.72,20.65 53.02,20.95 53.02,23.49 C4.1
POT_IN
  Top 0.406: R6.2 77.69,23.17 IC1.1 70.75,20.7 70.63,20.8 68.56,20.8 68.23,21.13 68.23,21.59 IC2.1
PWR_STIM
  Top 0.406: DUE.52 104.78,12.06 102.87,10.16 102.87,8.89 102.23,8.26 88.27,8.26 87,9.53 R13.2
PWR_SWITCH
  Top 0.406: DUE.22 107.61,50.16 106.56,51.2 106.56,53.41 107.56,54.41 112.56,54.41 112.97,54 112.97,53.2 113.18,52.99 R11.2
RESET
  Top 0.406: 137.8,33.94 R5.1 137.8,34.25 | OK5.4 132.08,32.98 136.84,32.98 137.8,33.94 | 137.8,33.94 137.83,33.94 138.76,33 142.8,33 X2.4
RESET_ARD
  Top 0.406: U5.9 118.77,32.41 118.75,32.38 118.75,31.11 118.11,30.48 113.03,30.48 DUE.37
RESET_INV
  Top 0.406: U5.8 119.43,35.47 121.36,37.41 123.8,37.41 OK5.1
RS232_RXD
  Top 0.406: U1.14 28.88,18.72 24.37,14.21 X3.3
RS232_TXD
  Top 0.406: U1.13 26.77,19.35 21.62,14.21 X3.2
SCL
  Top 0.406: DUE.SCL 100.97,52.07 97.79,48.89 97.79,31.75 93.34,27.3 69.85,27.3 69.22,26.67 69.22,26.03 68.58,25.4 68.55,25.43 IC2.6
SCLK
  Top 0.406: OK3.4 137.12,1.87 137.8,2.54 R3.1 139.29,4.93 140.76,6.4 140.76,24.41 142.29,25.93 X2.6
SCLK_ARD
  Top 0.406: U5.1 115.52,25.35 114.94,24.77 DUE.43
SCLK_INV
  Top 0.406: U5.2 116.2,26.9 116.2,22.86 119.38,19.69 119.38,10.16 119.41,10.16 122.56,7.01 123.77,7.01 OK3.1
SDA
  Top 0.406: DUE.SDA 98.42,51.43 97.16,50.16 97.16,32.38 92.71,27.94 68.58,27.94 67.65,27 IC2.7
STIM_OUT
  Top 0.406: J4.1 97.62,12.87 R9.2 Q2.3
STIM_REG_VIN-
  Top 0.406: Q3.3 V2.1 62.55,10.79 C20.1 C23.2
SW_REG_VIN-
  Top 0.406: C22.2 C12.1 120.41,49.84 121.56,51 123.39,51 V1.1 123.36,51.89 123.36,54.2 123.03,54.54 Q1.3
SYNC
  Top 0.406: OK4.4 136.53,41.91 137.8,43.18 | R4.1 137.8,43.18 | 137.8,43.18 139.7,41.27 139.7,37.78 141.95,35.53 X2.5
SYNC_ARD
  Top 0.406: U5.11 117.47,31.75 116.84,31.11 114.94,31.11 DUE.35
SYNC_INV
  Top 0.406: U5.10 118.14,35.59 120.97,38.41 120.97,45.8 122.17,47 123.81,47 OK4.1
TTL_RX
  Top 0.406: U1.12 47.95,20.02 49.53,21.59 49.53,23.49 54.61,28.57 92.08,28.57 96.52,33.02 96.52,50.16 95.89,50.8 DUE.RX1
TTL_TX
  Top 0.406: U1.11 47.32,20.65 47.62,20.95 47.62,22.86 53.98,29.21 91.44,29.21 95.89,33.66 95.89,48.89 93.34,51.43 DUE.TX1
V_STIM
  Top 0.406: Q2.2 R8.1 87.45,11.92 87.16,12.21 87.16,13.6 86.56,14.21 85.37,14.21 85.16,14.4 85.16,15.64 IC1.4 87.31,18.41 C14.2 R6.1
V_STIM_REF
  Top 0.406: IC1.3 71.81,16.13 C13.2 70.17,16.19 V2.4 | C15.1 C16.2 67.62,18.09 V2.4 | V2.4 66.04,20.32 66.04,23.49 66.67,24.13 IC2.4 68.29,24.13 69.56,25.41 70.41,25.41 C19.1 C18.2
(copper drawn outside any net)
  shapes: Bottom area x1071

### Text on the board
Bottom: JIMMY 2015
tPlace: SERIAL | I2C | 5V | GND | Tx | Rx | SDA | SCL | Pmark / in | ActiChamp / Triggers | SYNC | IND | Ex_3 | Ex_2 | Ex_1 | Freq | Stop | Start | Stim | Switch | GND | Sync | Phase MK / for stim | UCL EIT / SCOUSETOM V2 | Reset | RESET | DIN+ | GND | DIN- | PMARK | STIM / (3.3V) | Gnd | SCLK | DIN+ | STIM | Gnd | Keithley CS COMM | DIN- | SWITCH / NETWORK | 3v3 | 5V | GND | GND | STIM OUT | GND | GND | BYLAD | SCLK

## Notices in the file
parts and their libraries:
SparkFun-DiscreteSemi: Licensing: Creative Commons ShareAlike 4.0 International - https://creativecommons.org/licenses/by-sa/4.0
